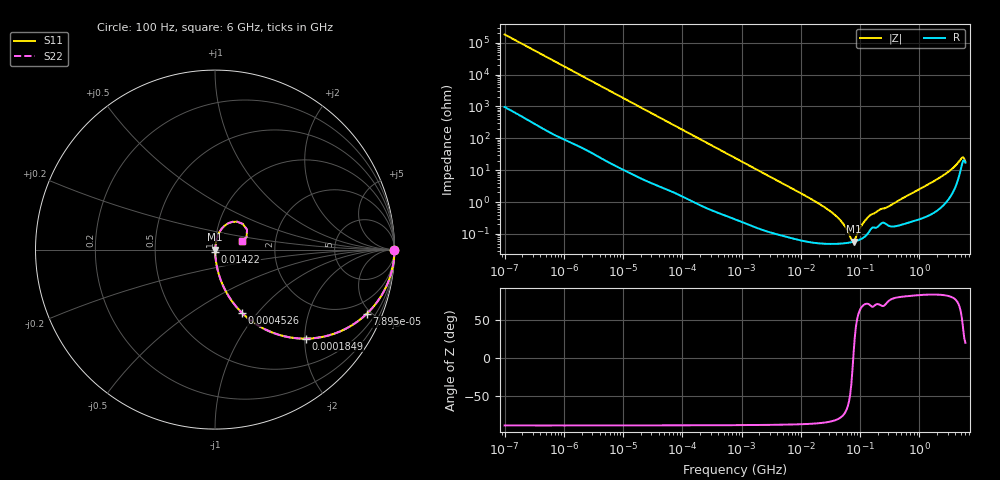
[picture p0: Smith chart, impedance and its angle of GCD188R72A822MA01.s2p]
!Murata Part Number: GCD188R72A822MA01
!These Parameters are Measured in Series Mode Connection
!Data Generated on Mar 13, 2026
!  o--ll--o
!Port1  Port2
!  o------o
!Operation Temp=25[degC], DC Bias Voltage=0[V]
!Freq. Start=100[Hz] Stop=6[GHz] 401[Steps]
# Hz S RI R 50
!Freq.(Hz) S11(Real) S11(Imag) S21(Real) S21(Imag) S12(Real) S12(Imag) S22(Real) S22(Imag)
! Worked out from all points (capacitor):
!   401 points, 100 Hz to 6 GHz, reference 50 ohm
!   read as one part in series: C = 8.73 nF near 109 Hz
!   lowest |Z| = 57.5 mohm at 77.97 MHz (marker M1)
!   series resonance near 76.82 MHz, so ESL is about 490 pH
!   S11 on the Smith chart (normalised r, x): 100 Hz: open; 78.95 kHz: 1.04, -4.72; 184.9 kHz: 1.02, -2.02; 452.6 kHz: 1.01, -0.83; 14.22 MHz: 1.00, -0.03; 6 GHz: 1.35, +0.13
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100  1 -0.000549  3.2e-06 0.000549  3.2e-06 0.000549  1 -0.000549
2008  0.9998 -0.0109  0.00018 0.0109  0.00018 0.0109  0.9998 -0.0109
12041  0.9954 -0.0648  0.00458 0.0648  0.00458 0.0648  0.9954 -0.0648
40335  0.9537 -0.2068  0.0463 0.2068  0.0463 0.2068  0.9537 -0.2068
78952  0.8459 -0.3572  0.1541 0.3572  0.1541 0.3572  0.8459 -0.3572
184852  0.5061 -0.4958  0.4939 0.4958  0.4939 0.4958  0.5061 -0.4958
452617  0.1496 -0.3516  0.8504 0.3516  0.8504 0.3516  0.1496 -0.3516
774597  0.0584 -0.2286  0.9416 0.2286  0.9416 0.2286  0.0584 -0.2286
2481164  0.00706 -0.0759  0.9929 0.0759  0.9929 0.0759  0.00706 -0.0759
1.422411e7  0.000719 -0.0131  0.9993 0.0131  0.9993 0.0131  0.000719 -0.0131
1.555665e7  0.000675 -0.0119  0.9993 0.0119  0.9993 0.0119  0.000675 -0.0119
4.165952e7  0.0005 -0.00328  0.9995 0.00328  0.9995 0.00328  0.0005 -0.00328
5.449875e7  0.000511 -0.00177  0.9995 0.00177  0.9995 0.00177  0.000511 -0.00177
7.129496e7  0.000549 -0.000378  0.9995 0.000378  0.9995 0.000378  0.000549 -0.000378
7.797396e7  0.00057 7.66e-05  0.9994 -7.66e-05  0.9994 -7.66e-05  0.00057 7.66e-05
1.066761e8  0.000709 0.00172  0.9993 -0.00172  0.9993 -0.00172  0.000709 0.00172
1.395531e8  0.00112 0.00331  0.9989 -0.00331  0.9989 -0.00331  0.00112 0.00331
3.124326e8  0.00182 0.00727  0.9982 -0.00727  0.9982 -0.00727  0.00182 0.00727
2.34314e9  0.0105 0.0611  0.9895 -0.0611  0.9895 -0.0611  0.0105 0.0611
3.8344e9  0.0363 0.1148  0.9637 -0.1148  0.9637 -0.1148  0.0363 0.1148
5.016141e9  0.1238 0.1554  0.8762 -0.1554  0.8762 -0.1554  0.1238 0.1554
6e9  0.1497 0.0457  0.8503 -0.0457  0.8503 -0.0457  0.1497 0.0457
